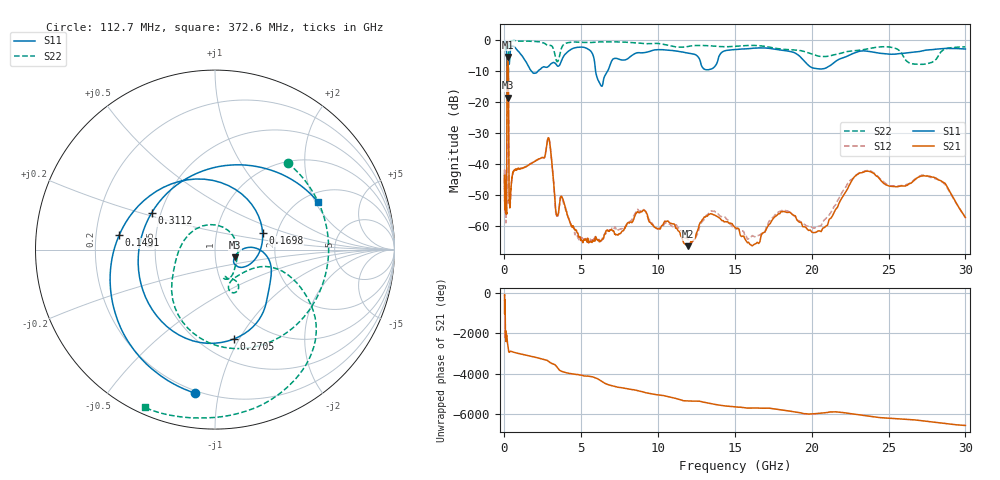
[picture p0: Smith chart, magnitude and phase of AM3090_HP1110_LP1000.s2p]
! Date/Time: Thu, Feb 28, 2019 2:09 PM
! Network Analyzer: Agilent Technologies E8364B Rev: A.07.50.67
! Sweep from 0.010 to 30.000 GHz, 1601 Points, Sweep Type: LOG
! Power Supply: 5.023 V, 0.002 A
# Hz S DB R 50
!freq MagS11 AngS11 MagS21 AngS21 MagS12 AngS12 MagS22 AngS22
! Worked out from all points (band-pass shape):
!   1601 points, 10 MHz to 30 GHz, reference 50 ohm
!   highest |S21| = -5.44 dB at 205.4 MHz (marker M1); lowest = -66.7 dB at 11.95 GHz (marker M2)
!   |S21| within 3 dB of the highest: 174.4 MHz to 247.2 MHz (72.81 MHz wide, 34.5 % of centre)
!   lowest |S11| = -18.6 dB at 210.6 MHz (marker M3), VSWR 1.27, Z = 62 - j5.4 ohm
!   |S11| at or under -10 dB: 166.4 MHz to 234.6 MHz (68.22 MHz wide, 34 % of centre); 1.746 GHz to 2.194 GHz (448.4 MHz wide, 22.8 % of centre); 5.93 GHz to 6.721 GHz (790.8 MHz wide, 12.5 % of centre)
!   |S22| runs from -18.0 to -0.1 dB; largest |S21 - S12| = 0.012
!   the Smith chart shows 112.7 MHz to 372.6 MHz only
!   S11 on the Smith chart (normalised r, x): 112.7 MHz: 0.18, -0.86; 149.1 MHz: 0.30, +0.07; 169.8 MHz: 1.68, +0.33; 270.5 MHz: 0.70, -0.95; 311.2 MHz: 0.44, +0.22; 372.6 MHz: 2.39, +2.11
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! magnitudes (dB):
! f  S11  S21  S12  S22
! 10 MHz  -0.3  -48.0  -42.1  -0.6
! 38.04 MHz  -0.3  -50.5  -49.9  -1.2
! 112.7 MHz  -1.8  -55.0  -53.1  -4.0
! 144.7 MHz  -4.5  -50.4  -49.3  -4.7
! 149.1 MHz  -5.4  -42.4  -42.1  -5.4
! 169.8 MHz  -11.0  -10.7  -10.7  -17.9
! 205.4 MHz  -18.1  -5.4  -5.4  -15.1
! 210.6 MHz  -18.6  -5.5  -5.4  -14.9
! 249.7 MHz  -8.5  -9.0  -9.0  -14.2
! 270.5 MHz  -5.9  -26.0  -26.0  -5.2
! 311.2 MHz  -7.8  -51.8  -51.0  -0.7
! 372.6 MHz  -4.0  -52.9  -52.6  -0.3
! 550.5 MHz  -2.0  -43.0  -43.3  -0.2
! 2.084 GHz  -10.6  -38.9  -38.8  -0.5
! 2.884 GHz  -8.4  -31.7  -31.7  -1.7
! 3.385 GHz  -8.0  -56.6  -56.7  -6.7
! 4.805 GHz  -2.3  -63.0  -64.2  -0.7
! 7.926 GHz  -6.3  -60.2  -59.7  -0.7
! 11.95 GHz  -4.2  -66.7  -64.4  -2.1
! 20.31 GHz  -9.2  -62.1  -60.3  -5.0
! 23.48 GHz  -3.5  -42.5  -42.4  -3.0
! 30 GHz  -2.9  -57.4  -57.4  -2.2
